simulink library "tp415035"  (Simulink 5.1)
undefined symbols (not defined in the file or in its folder): node_init, Retransmit, WLAN

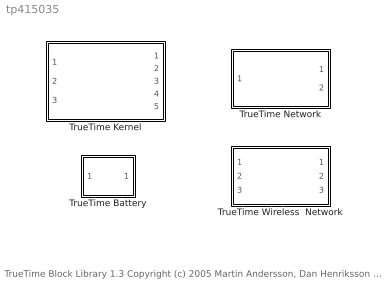
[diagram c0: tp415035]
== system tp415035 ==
  note: TrueTime Block Library 1.3 Copyright (c) 2005 Martin Andersson, Dan Henriksson and Anton Cervin Department of Automatic Control, Lund University, Sweden Please direct questions and bug reports to: truetime@control.lth.se
  TrueTime Battery : Subsystem  SimViewingDevice=off  mask{energy=1}
      mask prompts: energy "Watt seconds (Joule)"
  TrueTime Kernel : Subsystem  SimViewingDevice=off  mask{sfun=node_init, args=0, battery=off, clockdrift=0, clockoffset=0}
      mask prompts: sfun "Name of init function (MEX or MATLAB)"; args "Init function argument"; clockdrift "Clock drift"; clockoffset "Clock offset"
  TrueTime Network : Subsystem  SimViewingDevice=off  mask(Real-Time Network){nwtype=CSMA/CD (Ethernet), nwnbr=1, nnodes=2, rate=10000000, minsize=64, lossprob=0, bandwidths=[0.5 0.5], slotsize=64, schedule=0.5, memsize=10000, buftype=Common buffer, overflow=Retransmit}
      mask prompts: nwtype "Network type"; nwnbr "Network number"; nnodes "Number of nodes"; rate "Data rate (bits/s)"; minsize "Minimum frame size (bytes)"; lossprob "Loss probability (0-1)"; bandwidths "Bandwidth allocations"; slotsize "Slotsize (bytes)"; schedule "Cyclic schedule"; memsize "Total switch memory (bytes)"; buftype "Switch buffer type"; overflow "Switch overflow behavior"
  TrueTime Wireless  Network : Subsystem  SimViewingDevice=off  mask(Wireless Network){nwtype=802.11b (WLAN), nwnbr=1, nnodes=1, rate=800000, minsize=34, transpower=20, threshold=-48, pathloss=3.5, acktimeout=0.00004, retrylimit=5, error_threshold=0.03}
      mask prompts: nwtype "Network type"; nwnbr "Network Number"; nnodes "Number of nodes"; rate "Data rate (bits/s)"; minsize "Minimum frame size (bytes)"; transpower "Transmit power (dbm)"; threshold "Receiver signal threshold (dbm)"; pathloss "Pathloss exponent (1/distance^x)"; acktimeout "ACK timeout (s)"; retrylimit "Retry limit"; error_threshold "Error coding threshold"

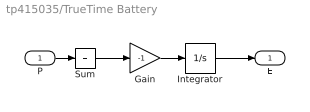
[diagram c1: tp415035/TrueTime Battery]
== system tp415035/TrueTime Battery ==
  P : Inport  Port=1  PortDimensions=-1  SampleTime=-1  DataType=auto
  Gain : Gain  Gain=-1  Multiplication=Element-wise(K.*u)  SaturateOnIntegerOverflow=on
  Integrator : Integrator  ExternalReset=none  InitialConditionSource=internal  InitialCondition=energy  LimitOutput=on  UpperSaturationLimit=energy  LowerSaturationLimit=0  ShowSaturationPort=off  ShowStatePort=off  AbsoluteTolerance=auto
  Sum : Sum  Inputs=1  SaturateOnIntegerOverflow=on
  E : Outport  Port=1
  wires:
  Integrator/1 -> E/1
  Gain/1 -> Integrator/1
  P/1 -> Sum/1
  Sum/1 -> Gain/1

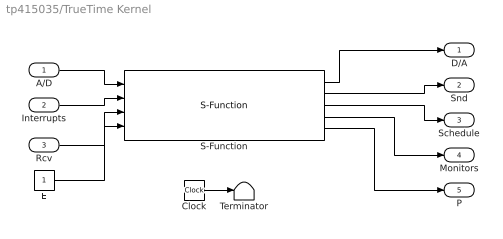
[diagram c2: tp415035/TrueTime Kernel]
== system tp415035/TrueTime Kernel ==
  A/D : Inport  Port=1  PortDimensions=-1  SampleTime=-1  DataType=auto
  Interrupts : Inport  Port=2  PortDimensions=-1  SampleTime=-1  DataType=auto
  Rcv : Inport  Port=3  PortDimensions=-1  SampleTime=-1  DataType=auto
  Clock : Clock
  E : Constant  Value=1
  S-Function : S-Function  FunctionName=eval(eval(['''sfunchk(''''' sfun ''''')''']))  Parameters=sfun, args, clockdrift, clockoffset  PortCounts=[]  SFunctionModules=''
  Terminator : Terminator
  D/A : Outport  Port=1
  Snd : Outport  Port=2
  Schedule : Outport  Port=3
  Monitors : Outport  Port=4
  P : Outport  Port=5
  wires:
  S-Function/5 -> P/1
  E/1 -> S-Function/4
  A/D/1 -> S-Function/1
  S-Function/2 -> Snd/1
  S-Function/1 -> D/A/1
  S-Function/3 -> Schedule/1
  S-Function/4 -> Monitors/1
  Interrupts/1 -> S-Function/2
  Rcv/1 -> S-Function/3
  Clock/1 -> Terminator/1

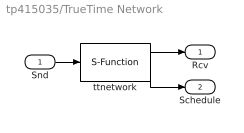
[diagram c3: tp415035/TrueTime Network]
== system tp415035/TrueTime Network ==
  Snd : Inport  Port=1  PortDimensions=-1  SampleTime=-1  DataType=auto
  ttnetwork : S-Function  FunctionName=ttnetwork  Parameters=nwtype,nwnbr,nnodes,rate,minsize,lossprob,bandwidths,slotsize,schedule,memsize,buftype,overflow  PortCounts=[]  SFunctionModules=''
  Rcv : Outport  Port=1
  Schedule : Outport  Port=2
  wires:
  ttnetwork/2 -> Schedule/1
  ttnetwork/1 -> Rcv/1
  Snd/1 -> ttnetwork/1

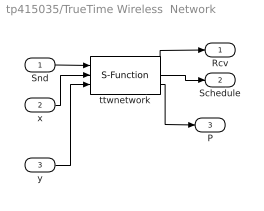
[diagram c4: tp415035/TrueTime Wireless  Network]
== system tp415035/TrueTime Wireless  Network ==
  Snd : Inport  Port=1  PortDimensions=-1  SampleTime=-1  DataType=auto
  x : Inport  Port=2  PortDimensions=-1  SampleTime=-1  DataType=auto
  y : Inport  Port=3  PortDimensions=-1  SampleTime=-1  DataType=auto
  ttwnetwork : S-Function  FunctionName=ttwnetwork  Parameters=nwtype,nwnbr,nnodes,rate,minsize,transpower,threshold,pathloss,acktimeout,retrylimit,error_threshold  PortCounts=[]  SFunctionModules=''
  Rcv : Outport  Port=1
  Schedule : Outport  Port=2
  P : Outport  Port=3
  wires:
  ttwnetwork/3 -> P/1
  Snd/1 -> ttwnetwork/1
  ttwnetwork/1 -> Rcv/1
  ttwnetwork/2 -> Schedule/1
  x/1 -> ttwnetwork/2
  y/1 -> ttwnetwork/3
